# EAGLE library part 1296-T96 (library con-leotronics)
1.27mm SINGLE ROW FEMALE SOCKET Source: http://www.leotronics.co.uk/Conexcon/Data%20Sheets/sec.%20A/1296ing.pdf
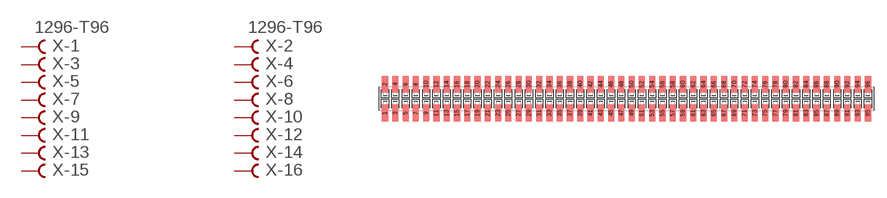
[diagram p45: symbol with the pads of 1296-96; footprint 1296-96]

Designator prefix X; gates -1=FVAL -2=FVAL -3=F -4=F -5=F -6=F -7=F -8=F -9=F -10=F -11=F -12=F -13=F -14=F -15=F -16=F -17=F -18=F -19=F -20=F -21=F -22=F -23=F -24=F -25=F -26=F -27=F -28=F -29=F -30=F -31=F -32=F -33=F -34=F -35=F -36=F -37=F -38=F -39=F -40=F -41=F -42=F -43=F -44=F -45=F -46=F -47=F -48=F -49=F -50=F -51=F -52=F -53=F -54=F -55=F -56=F -57=F -58=F -59=F -60=F -61=F -62=F -63=F -64=F -65=F -66=F -67=F -68=F -69=F -70=F -71=F -72=F -73=F -74=F -75=F -76=F -77=F -78=F -79=F -80=F -81=F -82=F -83=F -84=F -85=F -86=F -87=F -88=F -89=F -90=F -91=F -92=F -93=F -94=F -95=F -96=F

## 1296-T96 (OC_FARNELL: unknown; OC_NEWARK: unknown)  [1296-96]
1  -1:B  pas
2  -2:B  pas
3  -3:B  pas
4  -4:B  pas
5  -5:B  pas
6  -6:B  pas
7  -7:B  pas
8  -8:B  pas
9  -9:B  pas
10  -10:B  pas
11  -11:B  pas
12  -12:B  pas
13  -13:B  pas
14  -14:B  pas
15  -15:B  pas
16  -16:B  pas
17  -17:B  pas
18  -18:B  pas
19  -19:B  pas
20  -20:B  pas
21  -21:B  pas
22  -22:B  pas
23  -23:B  pas
24  -24:B  pas
25  -25:B  pas
26  -26:B  pas
27  -27:B  pas
28  -28:B  pas
29  -29:B  pas
30  -30:B  pas
31  -31:B  pas
32  -32:B  pas
33  -33:B  pas
34  -34:B  pas
35  -35:B  pas
36  -36:B  pas
37  -37:B  pas
38  -38:B  pas
39  -39:B  pas
40  -40:B  pas
41  -41:B  pas
42  -42:B  pas
43  -43:B  pas
44  -44:B  pas
45  -45:B  pas
46  -46:B  pas
47  -47:B  pas
48  -48:B  pas
49  -49:B  pas
50  -50:B  pas
51  -51:B  pas
52  -52:B  pas
53  -53:B  pas
54  -54:B  pas
55  -55:B  pas
56  -56:B  pas
57  -57:B  pas
58  -58:B  pas
59  -59:B  pas
60  -60:B  pas
61  -61:B  pas
62  -62:B  pas
63  -63:B  pas
64  -64:B  pas
65  -65:B  pas
66  -66:B  pas
67  -67:B  pas
68  -68:B  pas
69  -69:B  pas
70  -70:B  pas
71  -71:B  pas
72  -72:B  pas
73  -73:B  pas
74  -74:B  pas
75  -75:B  pas
76  -76:B  pas
77  -77:B  pas
78  -78:B  pas
79  -79:B  pas
80  -80:B  pas
81  -81:B  pas
82  -82:B  pas
83  -83:B  pas
84  -84:B  pas
85  -85:B  pas
86  -86:B  pas
87  -87:B  pas
88  -88:B  pas
89  -89:B  pas
90  -90:B  pas
91  -91:B  pas
92  -92:B  pas
93  -93:B  pas
94  -94:B  pas
95  -95:B  pas
96  -96:B  pas

## Footprint 1296-96 (pad centres in mm)
1.27mm SINGLE ROW FEMALE SOCKET Source: http://www.leotronics.co.uk/Conexcon/Data%20Sheets/sec.%20A/1296ing.pdf
smd 0.76 x 2.05: 1 -29.845,-1.78; 2 -29.845,1.78; 3 -28.575,-1.78; 4 -28.575,1.78; 5 -27.305,-1.78; 6 -27.305,1.78; 7 -26.035,-1.78; 8 -26.035,1.78; 9 -24.765,-1.78; 10 -24.765,1.78; 11 -23.495,-1.78; 12 -23.495,1.78; 13 -22.225,-1.78; 14 -22.225,1.78; 15 -20.955,-1.78; 16 -20.955,1.78; 17 -19.685,-1.78; 18 -19.685,1.78; 19 -18.415,-1.78; 20 -18.415,1.78; 21 -17.145,-1.78; 22 -17.145,1.78; 23 -15.875,-1.78; 24 -15.875,1.78; 25 -14.605,-1.78; 26 -14.605,1.78; 27 -13.335,-1.78; 28 -13.335,1.78; 29 -12.065,-1.78; 30 -12.065,1.78; 31 -10.795,-1.78; 32 -10.795,1.78; 33 -9.525,-1.78; 34 -9.525,1.78; 35 -8.255,-1.78; 36 -8.255,1.78; 37 -6.985,-1.78; 38 -6.985,1.78; 39 -5.715,-1.78; 40 -5.715,1.78; 41 -4.445,-1.78; 42 -4.445,1.78; 43 -3.175,-1.78; 44 -3.175,1.78; 45 -1.905,-1.78; 46 -1.905,1.78; 47 -0.635,-1.78; 48 -0.635,1.78; 49 0.635,-1.78; 50 0.635,1.78; 51 1.905,-1.78; 52 1.905,1.78; 53 3.175,-1.78; 54 3.175,1.78; 55 4.445,-1.78; 56 4.445,1.78; 57 5.715,-1.78; 58 5.715,1.78; 59 6.985,-1.78; 60 6.985,1.78; 61 8.255,-1.78; 62 8.255,1.78; 63 9.525,-1.78; 64 9.525,1.78; 65 10.795,-1.78; 66 10.795,1.78; 67 12.065,-1.78; 68 12.065,1.78; 69 13.335,-1.78; 70 13.335,1.78; 71 14.605,-1.78; 72 14.605,1.78; 73 15.875,-1.78; 74 15.875,1.78; 75 17.145,-1.78; 76 17.145,1.78; 77 18.415,-1.78; 78 18.415,1.78; 79 19.685,-1.78; 80 19.685,1.78; 81 20.955,-1.78; 82 20.955,1.78; 83 22.225,-1.78; 84 22.225,1.78; 85 23.495,-1.78; 86 23.495,1.78; 87 24.765,-1.78; 88 24.765,1.78; 89 26.035,-1.78; 90 26.035,1.78; 91 27.305,-1.78; 92 27.305,1.78; 93 28.575,-1.78; 94 28.575,1.78; 95 29.845,-1.78; 96 29.845,1.78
